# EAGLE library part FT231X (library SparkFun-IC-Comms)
FTDI FT231X Full Speed USB to Full-handshake UART This USB2.0 Full Speed IC offers a compact bridge to full handshake UART interfaces. The device is a UART, capable of operating up to 3MBaud, with low power consumption (8mA). The FT231X includes the complete FT-X series feature set and enables USB to be added into a system design quickly and easily over a UART interface. Datasheet SparkFun Products SparkFun RedBoard - Programmed with Arduino (DEV-12757) SparkFun XBee Explorer USB (WRL-11812) SparkFun XBee Explorer Dongle (WRL-11697) SparkFun Blynk Board - ESP8266 (WRL-13794) SparkFun ESP8266 Thing - Dev Board (WRL-13711) SparkFun Block for Intel® Edison - Base (DEV-13045) SparkFun RedStick (DEV-13741) SparkFun Beefy 3 - FTDI Basic Breakout (DEV-13746) SparkFun FT231X Breakout (BOB-11736)
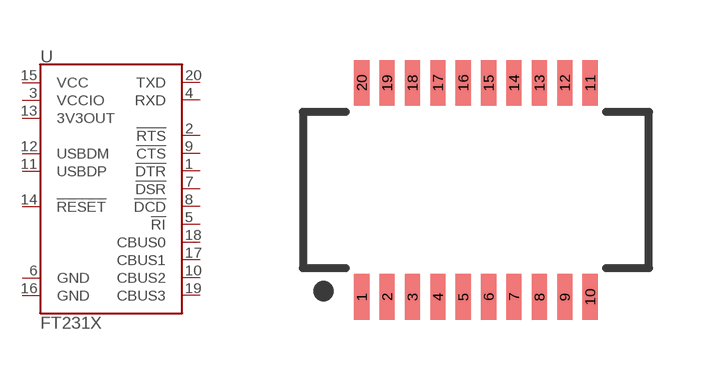
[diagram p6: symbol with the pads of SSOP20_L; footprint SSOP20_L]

Designator prefix U

## FT231XS (PROD_ID: IC-11524; VALUE: FT231XS)  [SSOP20_L]
1  !DTR
2  !RTS
3  VCCIO
4  RXD
5  !RI
6  GND
7  !DSR
8  !DCD
9  !CTS
10  CBUS2
11  USBDP
12  USBDM
13  3V3OUT
14  !RESET
15  VCC
16  GND
17  CBUS1
18  CBUS0
19  CBUS3
20  TXD

## Footprint SSOP20_L (pad centres in mm)
SSOP-20 -Long Version Specifications: Pin count:20 Example device(s): FT231X
smd 0.381 x 1.143: 1 -2.857,-2.68; 2 -2.223,-2.68; 3 -1.587,-2.68; 4 -0.953,-2.68; 5 -0.318,-2.68; 6 0.318,-2.68; 7 0.953,-2.68; 8 1.587,-2.68; 9 2.223,-2.68; 10 2.857,-2.68; 11 2.857,2.68; 12 2.223,2.68; 13 1.587,2.68; 14 0.953,2.68; 15 0.318,2.68; 16 -0.318,2.68; 17 -0.953,2.68; 18 -1.587,2.68; 19 -2.223,2.68; 20 -2.857,2.68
